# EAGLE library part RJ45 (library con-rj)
RJ45 RJ45 jacks side mounted http://www.tycoelectronics.com
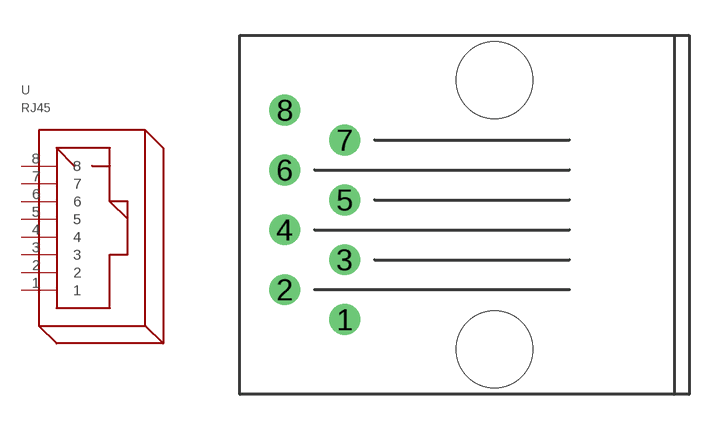
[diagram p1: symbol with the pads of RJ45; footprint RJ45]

Designator prefix -

## RJ45  [RJ45]
1  1
2  2
3  3
4  4
5  5
6  6
7  7
8  8

## Footprint RJ45 (pad centres in mm)
RJ45 RJ45 jacks side mounted http://www.tycoelectronics.com
drill 0.8: 1 -6.35,-4.445; 2 -8.89,-3.175; 3 -6.35,-1.905; 4 -8.89,-0.635; 5 -6.35,0.635; 6 -8.89,1.905; 7 -6.35,3.175; 8 -8.89,4.445
hole 3.25 at 0,-5.715
hole 3.25 at 0,5.715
